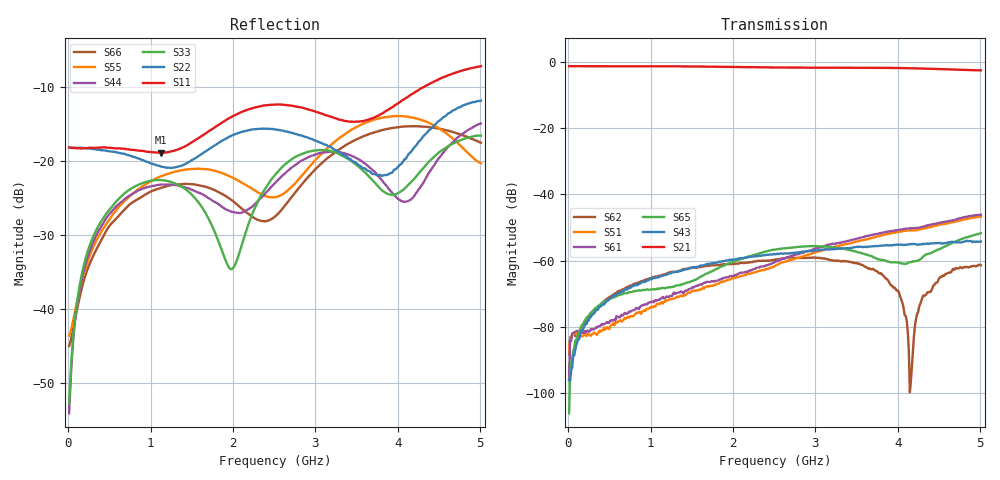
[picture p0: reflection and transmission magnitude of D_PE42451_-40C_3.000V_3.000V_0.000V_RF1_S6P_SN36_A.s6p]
! Device ID: PE42451
! Serial: 36
! Insertion: A
! Temp: -40C
! VDD: 3.000
! Control_Hi: 100.000
! Control_Lo: 0.000
! Logic State: RF1
! Port 1: RFC
! Port 2: RF1
! Port 3: RF2
! Port 4: RF3
! Port 5: RF4
! Port 6: RF5
! V1 = 3.00
! V2 = 0.00
! V3 = 0.00
! V4 = 0.00
! IDD: 1.326220e-05
#  Hz  S  RI  R  50
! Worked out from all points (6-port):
!   401 points, 10 MHz to 5.01 GHz, reference 50 ohm
!   strongest paths, dB at 10 MHz, 1.26 GHz, 2.51 GHz, 3.76 GHz, 5.01 GHz:
!     S21: -1.3, -1.3, -1.7, -1.8, -2.5
!     S43: -96.1, -63.5, -58.1, -55.6, -54.2
!     S65: -106.1, -67.9, -56.6, -59.6, -51.7
!     S61: -95.9, -70.6, -60.4, -51.9, -46.1
!     S51: -87.0, -71.5, -61.6, -52.6, -46.7
!     S62: -88.3, -63.4, -59.7, -63.5, -61.4
!   lowest |S11| = -18.8 dB at 1.123 GHz (marker M1), VSWR 1.26, Z = 57.3 - j9.96 ohm
!   |S11| at or under -10 dB: start of sweep to 4.309 GHz
